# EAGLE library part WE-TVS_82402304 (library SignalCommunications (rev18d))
TVS Diode Standard Series Characteristics Operating temperature: –55 ºC to +85 °C for 824 023 x; –55 ºC to +125 °C for 824 021/824 022 Very low clamping voltage High ESD withstand voltage Unidirectional or bidirectional protection RoHS, REACH and free of halogens Applications DC power supply Headsets and accessories PDAs Digital cameras MP3-Player Touch Panels ESD protection in accordance with EN 61000-4-2 – 8 kV contact discharge – 15 kV air discharge Updated by Dan Xu 2014-07-11 2014 (C) Wurth Elektronik
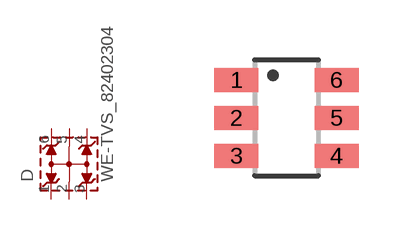
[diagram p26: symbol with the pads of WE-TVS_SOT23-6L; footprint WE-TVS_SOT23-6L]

Designator prefix D

## WE-TVS_82402304  [WE-TVS_SOT23-6L]
1  1
2  GND
3  2
4  3
5  GND
6  4

## Footprint WE-TVS_SOT23-6L (pad centres in mm)
TVS Diode Array WE-TVS
smd 1.1 x 0.6: 1 -1.25,0.95; 2 -1.25,0; 3 -1.25,-0.95; 4 1.25,-0.95; 5 1.25,0; 6 1.25,0.95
